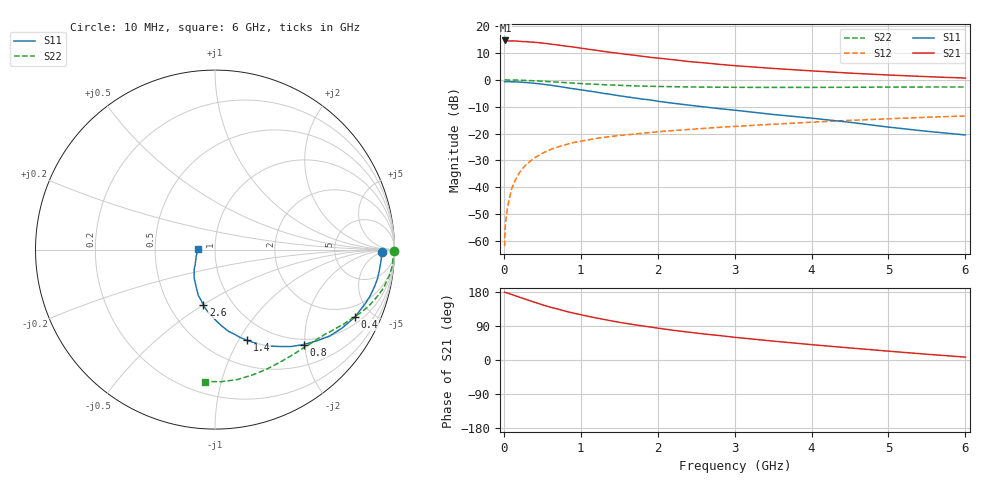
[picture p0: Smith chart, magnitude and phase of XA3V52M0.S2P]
! SIEMENS Discrete & RF Semiconductors
! BFY180
! Si NPN RF Bipolar Junction Transistor in MICRO-X
! VCE = 3.5 V  IC = 2 mA
! Common Emitter S-Parameters:  May  1997
# GHz  S  MA  R  50
!  f  S11  S21  S12  S22
! GHz  MAG  ANG  MAG  ANG  MAG  ANG  MAG  ANG
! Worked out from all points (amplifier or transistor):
!   36 points, 10 MHz to 6 GHz, reference 50 ohm
!   highest |S21| = 14.7 dB at 20 MHz (marker M1)
!   |S21| within 3 dB of that: start of sweep to 1.033 GHz
!   unconditionally stable (mu >= 1): 2.819 GHz to end of sweep
!   at 250 MHz: K = 0.13, MSG = 23.5 dB, |S12| = -32.8 dB
!   at 1.4 GHz: K = 0.68, MSG = 15.6 dB, |S12| = -21.1 dB
!   at 6 GHz: K = 1.06, MAG = 5.5 dB, |S12| = -13.4 dB
!   S11 on the Smith chart (normalised r, x): 10 MHz: 26, -4; 400 MHz: 1.32, -3.97; 800 MHz: 0.89, -1.97; 1.4 GHz: 0.77, -1.08; 2.6 GHz: 0.73, -0.50; 6 GHz: 0.83, +0.01
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0.01  0.9282 -0.7  5.31 179.0  0.0008 83.0  0.9955 -0.3
0.02  0.9292 -1.5  5.432 178.1  0.0021 89.4  0.9999 -0.7
0.05  0.9278 -3.3  5.328 176.5  0.0044 82.1  0.9958 -1.7
0.1  0.9237 -6.7  5.319 173.2  0.0093 85.1  0.9926 -3.3
0.15  0.9202 -10.0  5.314 169.5  0.0137 85.6  0.9929 -5.0
0.25  0.9028 -16.4  5.164 162.7  0.023 79.8  0.9829 -8.3
0.3  0.8912 -19.4  5.149 159.0  0.0273 77.5  0.9755 -9.8
0.4  0.8656 -25.7  5.017 152.3  0.0354 74.1  0.9632 -12.8
0.5  0.8326 -31.6  4.863 145.8  0.0429 70.1  0.9444 -15.6
0.6  0.7997 -37.1  4.667 139.5  0.05 67.1  0.927 -18.1
0.8  0.7233 -47.0  4.268 128.7  0.0619 61.9  0.8906 -22.7
0.9  0.6864 -51.9  4.109 124.1  0.0678 59.0  0.8728 -24.7
1.1  0.623 -59.7  3.722 115.2  0.0764 55.2  0.8406 -28.3
1.4  0.5351 -70.6  3.246 103.2  0.0885 50.6  0.803 -33.2
1.7  0.4617 -80.6  2.88 93.0  0.0979 47.1  0.7734 -37.4
2  0.4008 -88.4  2.553 84.1  0.1082 44.4  0.7569 -41.4
2.2  0.368 -93.4  2.38 78.5  0.1138 42.6  0.7479 -44.1
2.6  0.315 -102.0  2.082 68.7  0.1249 39.9  0.7345 -49.1
3.5  0.2273 -118.0  1.636 49.9  0.1494 33.9  0.7243 -60.3
4.5  0.1623 -135.7  1.338 31.8  0.1764 26.8  0.7292 -73.3
5.5  0.1104 -161.0  1.15 15.2  0.2014 19.2  0.7368 -87.3
6  0.0943 177.5  1.082 7.6  0.213 15.0  0.7371 -94.3
